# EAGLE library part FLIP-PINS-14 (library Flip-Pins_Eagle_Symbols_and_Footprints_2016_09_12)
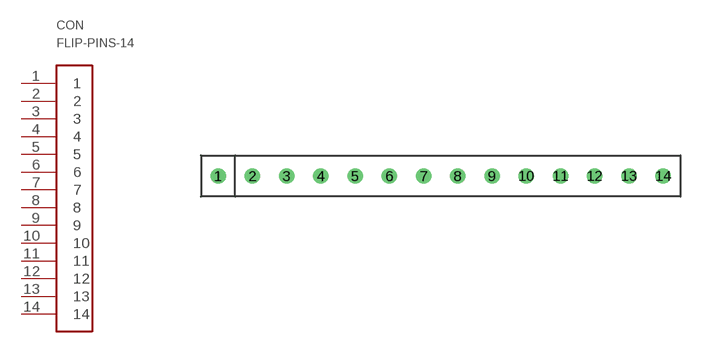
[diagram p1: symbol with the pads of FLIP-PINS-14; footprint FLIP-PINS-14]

Designator prefix CON

## FLIP-PINS-14  [FLIP-PINS-14]
1  1  pas
2  2  pas
3  3  pas
4  4  pas
5  5  pas
6  6  pas
7  7  pas
8  8  pas
9  9  pas
10  10  pas
11  11  pas
12  12  pas
13  13  pas
14  14  pas

## Footprint FLIP-PINS-14 (pad centres in mm)
drill 0.635 pad 1.016: 1 0,0; 2 2.54,0; 3 5.08,0; 4 7.62,0; 5 10.16,0; 6 12.7,0; 7 15.24,0; 8 17.78,0; 9 20.32,0; 10 22.86,0; 11 25.4,0; 12 27.94,0; 13 30.48,0; 14 33.02,0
